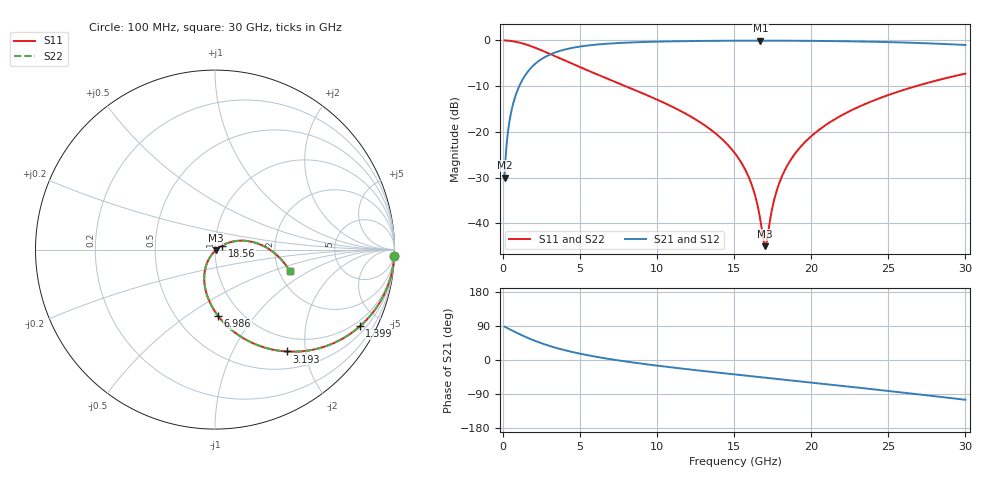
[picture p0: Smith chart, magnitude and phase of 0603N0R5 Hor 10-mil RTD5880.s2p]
# GHz S MA R 50
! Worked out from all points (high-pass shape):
!   3201 points, 100 MHz to 30 GHz, reference 50 ohm
!   highest |S21| = -0.05 dB at 16.69 GHz (marker M1); lowest = -30.0 dB at 100 MHz (marker M2)
!   |S21| within 3 dB of the highest: 3.066 GHz to end of sweep
!   lowest |S11| = -45.0 dB at 17.01 GHz (marker M3), VSWR 1.01, Z = 50.4 - j0.412 ohm
!   |S11| at or under -10 dB: 7.947 GHz to 26.79 GHz (18.84 GHz wide, 108 % of centre)
!   |S22| runs from -45.0 to 0.0 dB; largest |S21 - S12| = 0
!   S11 on the Smith chart (normalised r, x): 100 MHz: 1, -55; 1.399 GHz: 0.75, -3.88; 3.193 GHz: 0.76, -1.66; 6.986 GHz: 0.78, -0.67; 18.56 GHz: 1.08, +0.05; 30 GHz: 2.29, -0.68
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0.1  0.9995 -2.1  0.03168 87.9  0.03168 87.9  0.9995 -2.1
0.3429375  0.9941 -7.2  0.1081 82.8  0.1081 82.8  0.9941 -7.2
0.5671875  0.9842 -11.8  0.177 78.2  0.177 78.2  0.9842 -11.8
0.92225  0.9596 -18.9  0.281 71.1  0.281 71.1  0.9596 -18.9
1.398781  0.9133 -27.9  0.4066 62.0  0.4066 62.0  0.9133 -27.9
2.221031  0.8142 -41.7  0.5795 48.3  0.5795 48.3  0.8142 -41.7
3.192781  0.6938 -54.9  0.7186 35.0  0.7186 35.0  0.6938 -54.9
5.089563  0.5023 -73.9  0.8623 15.9  0.8623 15.9  0.5023 -73.9
6.986344  0.3688 -87.5  0.9265 2.1  0.9265 2.1  0.3688 -87.5
10.06978  0.2223 -104.2  0.971 -15.2  0.971 -15.2  0.2223 -104.2
13.12519  0.1167 -117.4  0.9884 -29.7  0.9884 -29.7  0.1167 -117.4
15.05  0.05815 -123.1  0.993 -38.2  0.993 -38.2  0.05815 -123.1
16.06847  0.0283 -121.7  0.994 -42.6  0.994 -42.6  0.0283 -121.7
16.41419  0.01844 -116.9  0.9942 -44.1  0.9942 -44.1  0.01844 -116.9
16.6945  0.01087 -104.7  0.9942 -45.3  0.9942 -45.3  0.01087 -104.7
17.01219  0.005623 -46.7  0.9941 -46.7  0.9941 -46.7  0.005623 -46.7
17.741  0.0223 25.1  0.9937 -49.8  0.9937 -49.8  0.0223 25.1
18.56325  0.04639 29.2  0.9926 -53.4  0.9926 -53.4  0.04639 29.2
20.03956  0.09097 26.2  0.9892 -59.8  0.9892 -59.8  0.09097 26.2
22.13256  0.1569 18.5  0.9803 -68.9  0.9803 -68.9  0.1569 18.5
25.01978  0.2536 6.4  0.9591 -81.8  0.9591 -81.8  0.2536 6.4
30  0.4335 -16.1  0.8916 -104.9  0.8916 -104.9  0.4335 -16.1
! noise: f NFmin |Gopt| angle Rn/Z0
0.1  0.0005884  0.9712  1.398  0.004633
3.417  0.004063  0.8126  10.73  0.004486
6.743  0.006793  0.7822  19.61  0.006218
10.06  0.009271  0.7655  28.5  0.007559
13.39  0.01167  0.7558  37.3  0.008692
16.7  0.01407  0.7508  45.89  0.009685
20.03  0.01655  0.7493  54.3  0.01058
23.35  0.01915  0.7507  62.46  0.01141
26.67  0.02194  0.7546  70.42  0.01217
30  0.025  0.7604  78.15  0.0129
